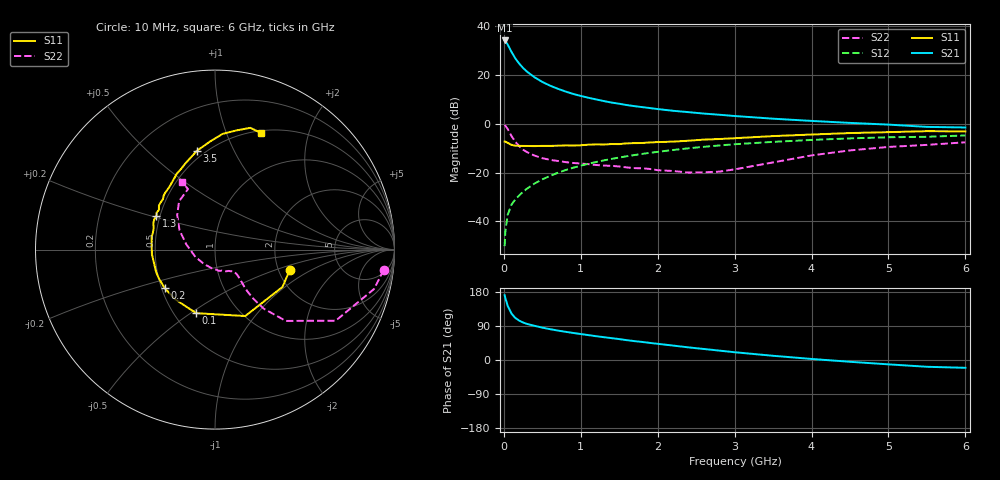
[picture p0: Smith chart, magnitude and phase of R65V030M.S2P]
! SIEMENS Small Signal Semiconductors
! BFR193
! Si NPN RF Bipolar Junction Transistor in SOT23
! VCE = 5 V  IC = 30 mA
! Common Emitter S-Parameters:  May  1996
# GHz  S  MA  R  50
!  f  S11  S21  S12  S22
! GHz  MAG  ANG  MAG  ANG  MAG  ANG  MAG  ANG
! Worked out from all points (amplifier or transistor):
!   36 points, 10 MHz to 6 GHz, reference 50 ohm
!   highest |S21| = 34.2 dB at 10 MHz (marker M1)
!   |S21| within 3 dB of that: start of sweep to 71.71 MHz
!   unconditionally stable (mu >= 1): 494.5 MHz to 1.899 GHz; 1.929 GHz to 2.007 GHz
!   at 250 MHz: K = 0.89, MSG = 25.4 dB, |S12| = -27.9 dB
!   at 1.4 GHz: K = 1.02, MAG = 10.6 dB, |S12| = -14.4 dB
!   at 6 GHz: K = 0.94, MSG = 1.6 dB, |S12| = -4.8 dB
!   lowest NFmin = 1.90 dB at 450 MHz
!   S11 on the Smith chart (normalised r, x): 10 MHz: 2.31, -0.64; 100 MHz: 0.64, -0.53; 200 MHz: 0.52, -0.25; 1.3 GHz: 0.48, +0.21; 3.5 GHz: 0.45, +0.73; 6 GHz: 0.52, +1.33
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0.01  0.4322 -15.1  51.07 171.2  0.0031 83.1  0.9467 -6.9
0.02  0.4296 -29.0  49.58 163.0  0.0063 82.1  0.9129 -13.9
0.05  0.4068 -65.5  42.09 143.0  0.0136 69.5  0.7805 -30.5
0.1  0.3692 -106.4  29.66 122.3  0.0221 64.9  0.56 -45.2
0.15  0.3551 -128.7  21.8 110.8  0.0282 65.4  0.426 -50.5
0.2  0.3529 -142.7  17.12 103.9  0.0341 67.4  0.3476 -52.0
0.25  0.3516 -152.7  13.94 99.0  0.0404 68.5  0.2948 -52.2
0.3  0.3512 -159.0  11.75 95.3  0.0466 69.8  0.2631 -51.7
0.4  0.3483 -168.8  8.964 90.1  0.0598 71.3  0.2225 -50.1
0.5  0.3526 -176.0  7.216 85.4  0.0725 71.5  0.1971 -48.9
0.6  0.3525 178.6  6.053 81.4  0.0853 71.3  0.1827 -48.6
0.8  0.3605 168.7  4.597 74.5  0.1123 70.1  0.1641 -49.7
0.9  0.3582 165.0  4.099 71.4  0.1255 69.1  0.1575 -50.1
1.1  0.373 157.3  3.414 65.7  0.1518 67.0  0.1488 -54.2
1.3  0.376 150.2  2.922 60.2  0.1778 64.7  0.1393 -58.5
1.7  0.4012 138.7  2.295 49.8  0.2289 59.4  0.1233 -71.7
2.2  0.4311 126.3  1.848 38.1  0.2906 52.3  0.1077 -97.3
2.8  0.4874 112.8  1.533 24.8  0.3595 43.3  0.1045 -144.9
3.5  0.5595 100.4  1.272 11.1  0.426 32.4  0.1616 170.0
4.5  0.6457 86.3  1.043 -4.7  0.5023 18.3  0.2847 137.7
5.5  0.7065 73.8  0.864 -17.9  0.5412 4.4  0.3694 114.0
6  0.6985 68.5  0.84 -20.6  0.5766 0.3  0.4178 116.0
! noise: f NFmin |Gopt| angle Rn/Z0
0.45  1.9  0.4  180  0.09
0.9  1.95  0.43  -173  0.11
1.8  2.4  0.58  -144  0.24
